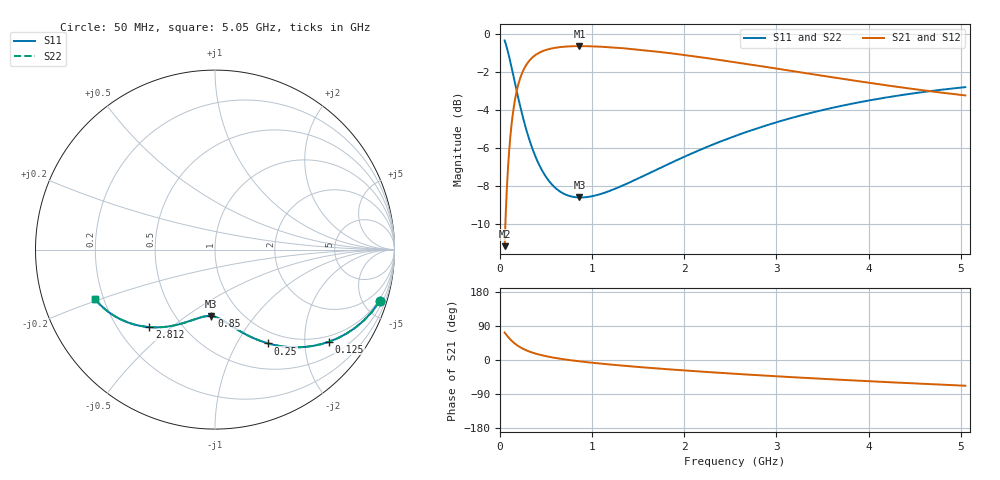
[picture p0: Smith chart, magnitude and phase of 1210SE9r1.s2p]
! AVX Thin Film Operation		Date: August 2001
! Description: Accu-P® Series, Thin Film, SMD, RF Capacitor
! Part Number: 12101J9R1BBT
! 50 MHz  -  5.05 GHz
! Serial Measurements
# mhz S db R 50
!	S11		S21		S12		S22
!	dB	Phase	dB	Phase	dB	Phase	dB	Phase
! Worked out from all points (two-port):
!   401 points, 50 MHz to 5.05 GHz, reference 50 ohm
!   highest |S21| = -0.64 dB at 862.5 MHz (marker M1); lowest = -11.2 dB at 50 MHz (marker M2)
!   |S21| within 3 dB of the highest: 156.8 MHz to end of sweep
!   lowest |S11| = -8.6 dB at 862.5 MHz (marker M3), VSWR 2.18, Z = 36.5 - j31.3 ohm
!   |S11| at or under -10 dB: nowhere
!   |S22| runs from -8.6 to -0.3 dB; largest |S21 - S12| = 0
!   S11 on the Smith chart (normalised r, x): 50 MHz: 0.84, -6.39; 125 MHz: 0.84, -2.59; 250 MHz: 0.83, -1.36; 850 MHz: 0.73, -0.63; 2.812 GHz: 0.33, -0.42; 5.05 GHz: 0.17, -0.19
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50  -0.34 -17.5  -11.19 72.5  -11.19 72.5  -0.34 -17.5
75  -0.73 -25.4  -8.10 64.6  -8.10 64.6  -0.73 -25.4
100  -1.22 -32.6  -6.13 57.4  -6.13 57.4  -1.22 -32.6
125  -1.75 -38.9  -4.79 51.1  -4.79 51.1  -1.75 -38.9
150  -2.31 -44.4  -3.85 45.6  -3.85 45.6  -2.31 -44.4
187.5  -3.15 -51.4  -2.88 38.6  -2.88 38.6  -3.15 -51.4
250  -4.42 -60.4  -1.95 29.6  -1.95 29.6  -4.42 -60.4
287.5  -5.09 -64.7  -1.61 25.3  -1.61 25.3  -5.09 -64.7
337.5  -5.86 -69.3  -1.31 20.6  -1.31 20.6  -5.86 -69.3
462.5  -7.25 -77.9  -0.91 12.1  -0.91 12.1  -7.25 -77.9
637.5  -8.26 -86.0  -0.70 3.9  -0.70 3.9  -8.26 -86.0
850  -8.62 -93.1  -0.64 -3.2  -0.64 -3.2  -8.62 -93.1
862.5  -8.62 -93.5  -0.64 -3.5  -0.64 -3.5  -8.62 -93.5
887.5  -8.62 -94.2  -0.64 -4.2  -0.64 -4.2  -8.62 -94.2
1262.5  -8.14 -103.4  -0.73 -13.4  -0.73 -13.4  -8.14 -103.4
1725  -7.10 -112.6  -0.95 -22.7  -0.95 -22.7  -7.10 -112.6
2112.5  -6.24 -119.4  -1.19 -29.4  -1.19 -29.4  -6.24 -119.4
2550  -5.38 -126.4  -1.49 -36.4  -1.49 -36.4  -5.38 -126.4
2812.5  -4.94 -130.3  -1.69 -40.3  -1.69 -40.3  -4.94 -130.3
3387.5  -4.15 -138.2  -2.12 -48.2  -2.12 -48.2  -4.15 -138.2
4225  -3.32 -148.6  -2.73 -58.6  -2.73 -58.6  -3.32 -148.6
5050  -2.81 -157.9  -3.24 -67.9  -3.24 -67.9  -2.81 -157.9
